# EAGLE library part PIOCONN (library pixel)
CONNECTOR 68-pin 1.27mm (.050 inch) pitch SCSI+ unshielded receptacle right angle all plastic
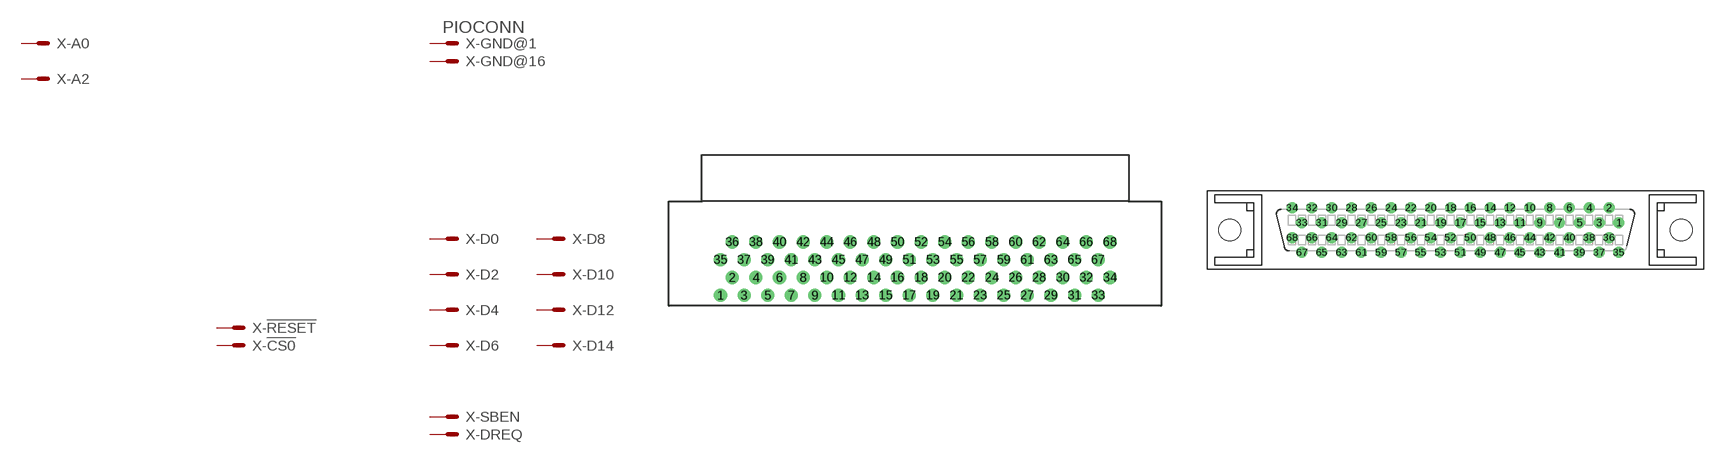
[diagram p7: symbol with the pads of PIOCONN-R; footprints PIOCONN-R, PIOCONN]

Designator prefix X; gates -GND@1=MV -!RESET=M -DREQ=M -!CS0=M -SBEN=M -D0=M -D2=M -D4=M -D6=M -D8=M -D10=M -D12=M -D14=M -A0=M -A2=M -GND@16=M -VCC33@17=M -VCC8@18=M -GND@19=M -A4=M -A6=M -A8=M -A10=M -A12=M -A14=M -A16=M -A18=M -A20=M -A22=M -!RD=M -!IN2=M -CLK=M -BCLK=M -GND@34=M -GND@35=M -DACK=M -!IN10=M -!WR2=M -!CS2=M -D1=M -D3=M -D5=M -D7=M -D9=M -D11=M -D13=M -D15=M -A1=M -A3=M -GND@50=M -VCC33@51=M -VCC8@52=M -GND@53=M -A5=M -A7=M -A9=M -A11=M -A13=M -A15=M -A17=M -A19=M -A21=M -A23=M -!WR=M -!CS5=M -LRCLK=M -SDIN=M -GND@68=M

## PIOCONNPIOCONN-R (MF: MOLEX; OC_FARNELL: unknown; OC_NEWARK: unknown)  [PIOCONN-R]
1  -GND@1:S  pas
2  -!RESET:S  pas
3  -DREQ:S  pas
4  -!CS0:S  pas
5  -SBEN:S  pas
6  -D0:S  pas
7  -D2:S  pas
8  -D4:S  pas
9  -D6:S  pas
10  -D8:S  pas
11  -D10:S  pas
12  -D12:S  pas
13  -D14:S  pas
14  -A0:S  pas
15  -A2:S  pas
16  -GND@16:S  pas
17  -VCC33@17:S  pas
18  -VCC8@18:S  pas
19  -GND@19:S  pas
20  -A4:S  pas
21  -A6:S  pas
22  -A8:S  pas
23  -A10:S  pas
24  -A12:S  pas
25  -A14:S  pas
26  -A16:S  pas
27  -A18:S  pas
28  -A20:S  pas
29  -A22:S  pas
30  -!RD:S  pas
31  -!IN2:S  pas
32  -CLK:S  pas
33  -BCLK:S  pas
34  -GND@34:S  pas
35  -GND@35:S  pas
36  -DACK:S  pas
37  -!IN10:S  pas
38  -!WR2:S  pas
39  -!CS2:S  pas
40  -D1:S  pas
41  -D3:S  pas
42  -D5:S  pas
43  -D7:S  pas
44  -D9:S  pas
45  -D11:S  pas
46  -D13:S  pas
47  -D15:S  pas
48  -A1:S  pas
49  -A3:S  pas
50  -GND@50:S  pas
51  -VCC33@51:S  pas
52  -VCC8@52:S  pas
53  -GND@53:S  pas
54  -A5:S  pas
55  -A7:S  pas
56  -A9:S  pas
57  -A11:S  pas
58  -A13:S  pas
59  -A15:S  pas
60  -A17:S  pas
61  -A19:S  pas
62  -A21:S  pas
63  -A23:S  pas
64  -!WR:S  pas
65  -!CS5:S  pas
66  -LRCLK:S  pas
67  -SDIN:S  pas
68  -GND@68:S  pas

## PIOCONNPIOCONN-S  [PIOCONN]
Pads as for PIOCONN-R

## Footprint PIOCONN-R (pad centres in mm)
drill 0.9 pad 1.27: 1 -20.955,-5.73; 2 -19.685,-3.82; 3 -18.415,-5.73; 4 -17.145,-3.82; 5 -15.875,-5.73; 6 -14.605,-3.82; 7 -13.335,-5.73; 8 -12.065,-3.82; 9 -10.795,-5.73; 10 -9.525,-3.82; 11 -8.255,-5.73; 12 -6.985,-3.82; 13 -5.715,-5.73; 14 -4.445,-3.82; 15 -3.175,-5.73; 16 -1.905,-3.82; 17 -0.635,-5.73; 18 0.635,-3.82; 19 1.905,-5.73; 20 3.175,-3.82; 21 4.445,-5.73; 22 5.715,-3.82; 23 6.985,-5.73; 24 8.255,-3.82; 25 9.525,-5.73; 26 10.795,-3.82; 27 12.065,-5.73; 28 13.335,-3.82; 29 14.605,-5.73; 30 15.875,-3.82; 31 17.145,-5.73; 32 18.415,-3.82; 33 19.685,-5.73; 34 20.955,-3.82; 35 -20.955,-1.91; 36 -19.685,0; 37 -18.415,-1.91; 38 -17.145,0; 39 -15.875,-1.91; 40 -14.605,0; 41 -13.335,-1.91; 42 -12.065,0; 43 -10.795,-1.91; 44 -9.525,0; 45 -8.255,-1.91; 46 -6.985,0; 47 -5.715,-1.91; 48 -4.445,0; 49 -3.175,-1.91; 50 -1.905,0; 51 -0.635,-1.91; 52 0.635,0; 53 1.905,-1.91; 54 3.175,0; 55 4.445,-1.91; 56 5.715,0; 57 6.985,-1.91; 58 8.255,0; 59 9.525,-1.91; 60 10.795,0; 61 12.065,-1.91; 62 13.335,0; 63 14.605,-1.91; 64 15.875,0; 65 17.145,-1.91; 66 18.415,0; 67 19.685,-1.91; 68 20.955,0

## Footprint PIOCONN (pad centres in mm)
TE CONNECTIVITY / AMP - BUCHSE, SCSI, VERTIKAL, 68 Source: Data sheet
drill 0.9 pad 1.27: 1 20.955,0.953; 2 19.685,2.863; 3 18.415,0.953; 4 17.145,2.863; 5 15.875,0.953; 6 14.605,2.863; 7 13.335,0.953; 8 12.065,2.863; 9 10.795,0.953; 10 9.525,2.863; 11 8.255,0.953; 12 6.985,2.863; 13 5.715,0.953; 14 4.445,2.863; 15 3.175,0.953; 16 1.905,2.863; 17 0.635,0.953; 18 -0.635,2.863; 19 -1.905,0.953; 20 -3.175,2.863; 21 -4.445,0.953; 22 -5.715,2.863; 23 -6.985,0.953; 24 -8.255,2.863; 25 -9.525,0.953; 26 -10.795,2.863; 27 -12.065,0.953; 28 -13.335,2.863; 29 -14.605,0.953; 30 -15.875,2.863; 31 -17.145,0.953; 32 -18.415,2.863; 33 -19.685,0.953; 34 -20.955,2.863; 35 20.955,-2.867; 36 19.685,-0.957; 37 18.415,-2.867; 38 17.145,-0.957; 39 15.875,-2.867; 40 14.605,-0.957; 41 13.335,-2.867; 42 12.065,-0.957; 43 10.795,-2.867; 44 9.525,-0.957; 45 8.255,-2.867; 46 6.985,-0.957; 47 5.715,-2.867; 48 4.445,-0.957; 49 3.175,-2.867; 50 1.905,-0.957; 51 0.635,-2.867; 52 -0.635,-0.957; 53 -1.905,-2.867; 54 -3.175,-0.957; 55 -4.445,-2.867; 56 -5.715,-0.957; 57 -6.985,-2.867; 58 -8.255,-0.957; 59 -9.525,-2.867; 60 -10.795,-0.957; 61 -12.065,-2.867; 62 -13.335,-0.957; 63 -14.605,-2.867; 64 -15.875,-0.957; 65 -17.145,-2.867; 66 -18.415,-0.957; 67 -19.685,-2.867; 68 -20.955,-0.957
hole 2.8 at -28.955,0
hole 2.8 at 28.955,0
